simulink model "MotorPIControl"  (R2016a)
settings: Solver=VariableStepAuto  StartTime=0.0  StopTime=Tf  RelTol=1e-7  AbsTol=1e-6
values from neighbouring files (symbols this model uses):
  d = 0    [Section4p2_DCMotorOpenLoop.m]    (also in Section4p3_DCMotorPControl.m; Section4p4_DCMotorPIControl.m; Section4p5_RocketPDControl.m = -0.01; Section4p6_PIDSecondOrder.m = 2)
  Gden = [1 a0]    [Section4p2_DCMotorOpenLoop.m]    (also in Section4p3_DCMotorPControl.m = [J*L (J*R+b*L) (Kt*Ke+b*R)]; Section4p4_DCMotorPIControl.m; Section4p5_RocketPDControl.m = [1 a1 a0]; Section4p6_PIDSecondOrder.m = [1 a1 a0])
  Gnum = b0    (= 766.8)    [Section4p2_DCMotorOpenLoop.m]    (also in Section4p3_DCMotorPControl.m = 0.00122680374957; Section4p4_DCMotorPIControl.m; Section4p5_RocketPDControl.m = 6.32; Section4p6_PIDSecondOrder.m = 17)
  Ki = Kp/2    (= 0.001)    [Section4p4_DCMotorPIControl.m]    (also in Section4p6_PIDSecondOrder.m = 15.006002401; Section4p6_PIFirstOrder.m = 10.8843537415)
  Kp = 16    [Section4p3_DCMotorPControl.m]    (also in Section4p4_DCMotorPIControl.m = 0.002; Section4p5_RocketPDControl.m = (wn^2-a0)/b0; Section4p6_PIDSecondOrder.m = 4.94237695078; Section4p6_PIFirstOrder.m = 2)
  r = 1000    [Section4p2_DCMotorOpenLoop.m]    (also in Section4p3_DCMotorPControl.m; Section4p4_DCMotorPIControl.m; Section4p5_RocketPDControl.m = 0.1; Section4p6_PIDSecondOrder.m = 4)
  Tf = 5    [Section4p2_DCMotorOpenLoop.m]    (also in Section4p3_DCMotorPControl.m = 0.005; Section4p4_DCMotorPIControl.m = 10; Section4p5_RocketPDControl.m = 10; Section4p6_PIDSecondOrder.m = 4)
  ulim = inf    [Section4p3_DCMotorPControl.m]    (also in Section4p4_DCMotorPIControl.m; Section4p5_RocketPDControl.m)

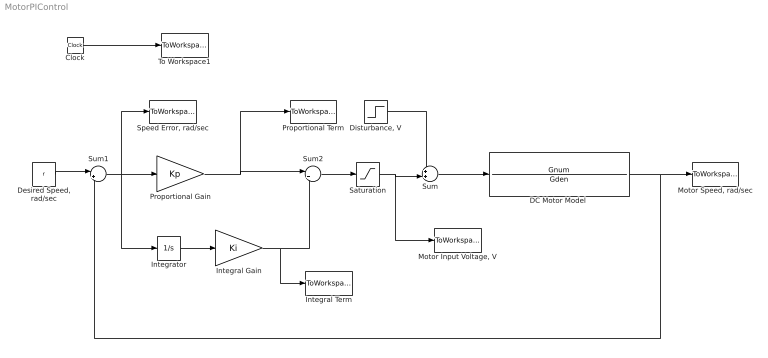
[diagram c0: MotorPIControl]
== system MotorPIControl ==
  Clock : Clock
  "DC Motor Model " : TransferFcn  Numerator=Gnum  Denominator=Gden
  "Desired Speed, rad/sec" : Constant  Value=r
  "Disturbance, V" : Step  Time=Tf/2  After=d  SampleTime=0
  Integral Term : ToWorkspace  VariableName=ui  SampleTime=-1
  Integral Gain : Gain  Gain=Ki
  Integrator : Integrator
  "Motor Input Voltage, V" : ToWorkspace  VariableName=u  SampleTime=-1
  "Motor Speed, rad/sec" : ToWorkspace  VariableName=y  SampleTime=-1
  Proportional Gain : Gain  Gain=Kp
  Proportional Term : ToWorkspace  VariableName=up  SampleTime=-1
  Saturation : Saturate  UpperLimit=ulim  LowerLimit=-ulim
  "Speed Error, rad/sec" : ToWorkspace  VariableName=e  SampleTime=-1
  Sum : Sum  Inputs=++|
  Sum1 : Sum  Inputs=|+-
  Sum2 : Sum  Inputs=|++
  To Workspace1 : ToWorkspace  VariableName=t  SampleTime=-1
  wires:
  Clock/1 -> To Workspace1/1
  "Disturbance, V"/1 -> Sum/1
  Sum/1 -> "DC Motor Model "/1
  "DC Motor Model "/1 -> Sum1/2, "Motor Speed, rad/sec"/1
  "Desired Speed, rad/sec"/1 -> Sum1/1
  Sum1/1 -> Integrator/1, Proportional Gain/1, "Speed Error, rad/sec"/1
  Saturation/1 -> Sum/2, "Motor Input Voltage, V"/1
  Integrator/1 -> Integral Gain/1
  Sum2/1 -> Saturation/1
  Integral Gain/1 -> Integral Term/1, Sum2/2
  Proportional Gain/1 -> Proportional Term/1, Sum2/1
